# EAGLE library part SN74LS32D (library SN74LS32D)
Texas Instruments SN74LS32D, OR Quad 2 Input OR, 4.75 5.25 V, 14-Pin SOIC Source: Datasheet
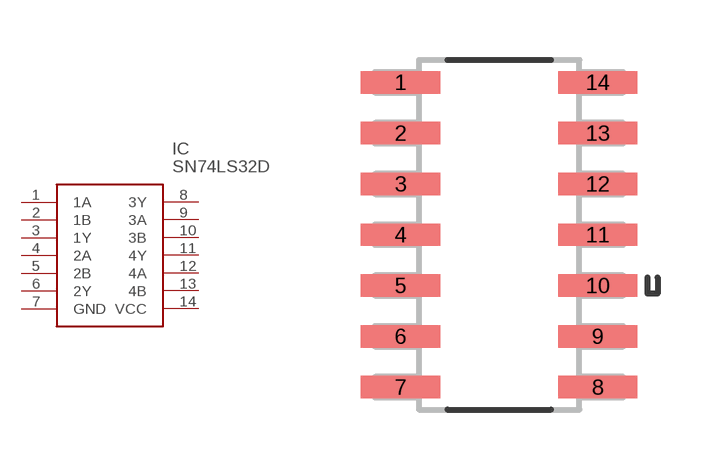
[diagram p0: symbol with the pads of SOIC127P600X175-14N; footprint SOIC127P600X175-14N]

Designator prefix IC

## SN74LS32D (Description: Texas Instruments SN74LS32D, OR Quad 2 Input OR, 4.75 5.25 V, 14-Pin SOIC; Height: mm; Manufacturer_Name: Texas Instruments; Manufacturer_Part_Number: SN74LS32D; Mouser_Part_Number: 595-SN74LS32D; Mouser_Price-Stock: https://www.mouser.com/Search/Refine.aspx?Keyword=595-SN74LS32D; RS_Part_Number: 1792177; RS_Price-Stock: http://uk.rs-online.com/web/p/products/1792177)  [SOIC127P600X175-14N]
1  1A
2  1B
3  1Y
4  2A
5  2B
6  2Y
7  GND
8  3Y
9  3A
10  3B
11  4Y
12  4A
13  4B
14  VCC

## Footprint SOIC127P600X175-14N (pad centres in mm)
SOIC127P600X175-14N
smd 1.981 x 0.559: 1 -2.464,3.81; 2 -2.464,2.54; 3 -2.464,1.27; 4 -2.464,0; 5 -2.464,-1.27; 6 -2.464,-2.54; 7 -2.464,-3.81; 8 2.464,-3.81; 9 2.464,-2.54; 10 2.464,-1.27; 11 2.464,0; 12 2.464,1.27; 13 2.464,2.54; 14 2.464,3.81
